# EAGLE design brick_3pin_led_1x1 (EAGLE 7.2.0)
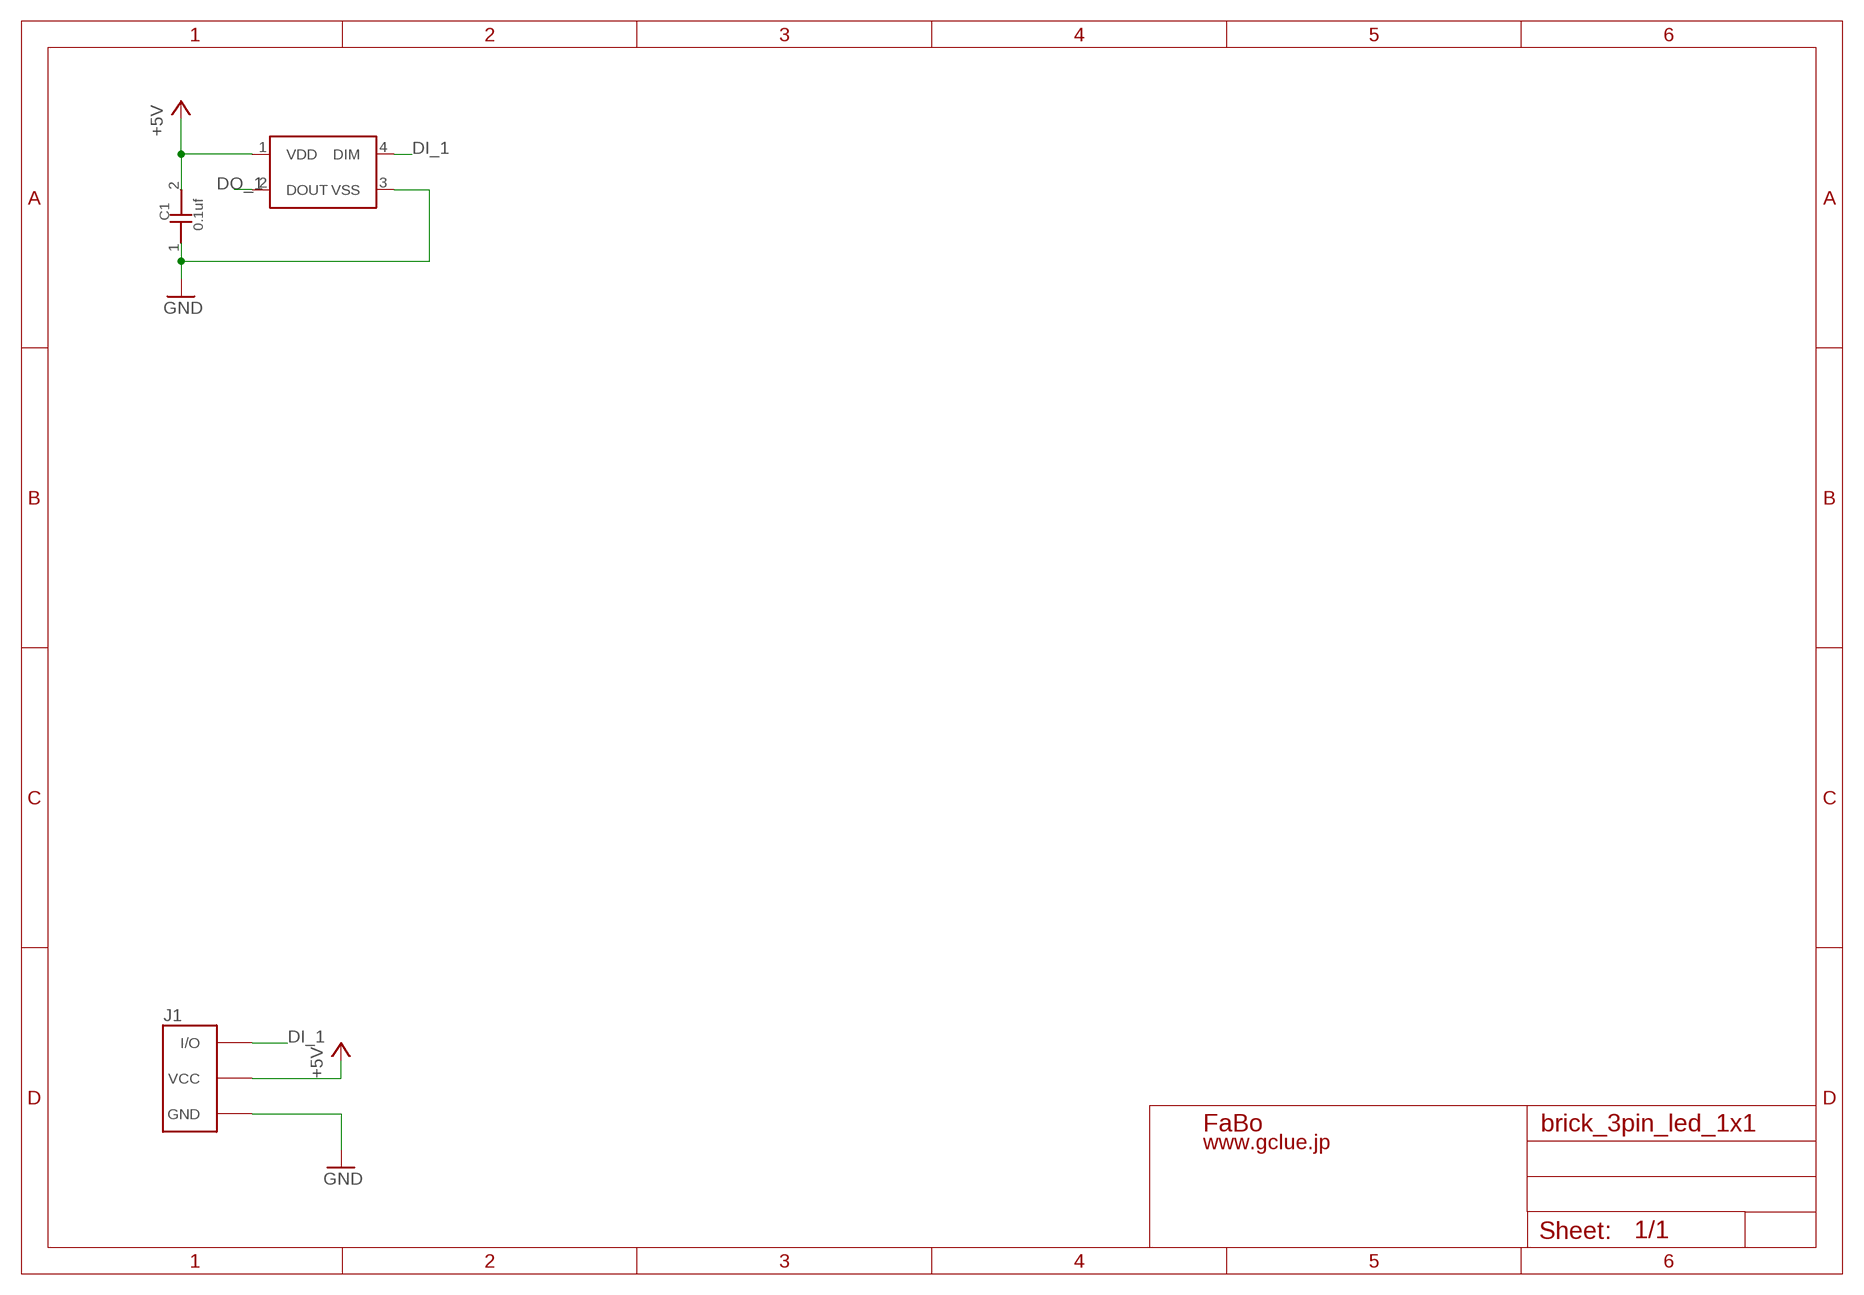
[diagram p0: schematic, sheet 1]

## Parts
C1  0.1uf  CAPACITOR0603  [0603]
J1  BRICK_3PIN  [BRICK_3PIN]
LED1  WS2818B  [WS2818B]

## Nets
+5V: C1.2 J1.VCC LED1.1(VDD)
DI_1: J1.IN/OUT(I/O) LED1.4(DIM)
DO_1: LED1.2(DOUT)
GND: C1.1 J1.GND LED1.3(VSS)

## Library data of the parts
C1 = GClue-Capacitor:CAPACITOR
J1 = GClue:BRICK_3PIN: FaBo Brick 3pin
LED1 = GClue-LED:WS2818B

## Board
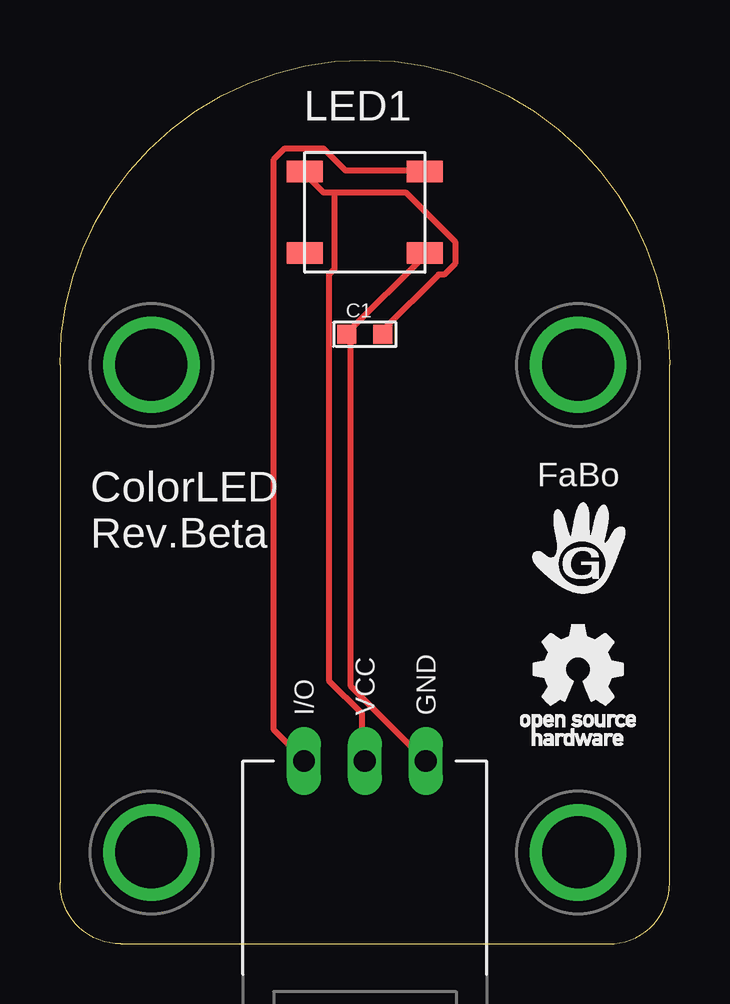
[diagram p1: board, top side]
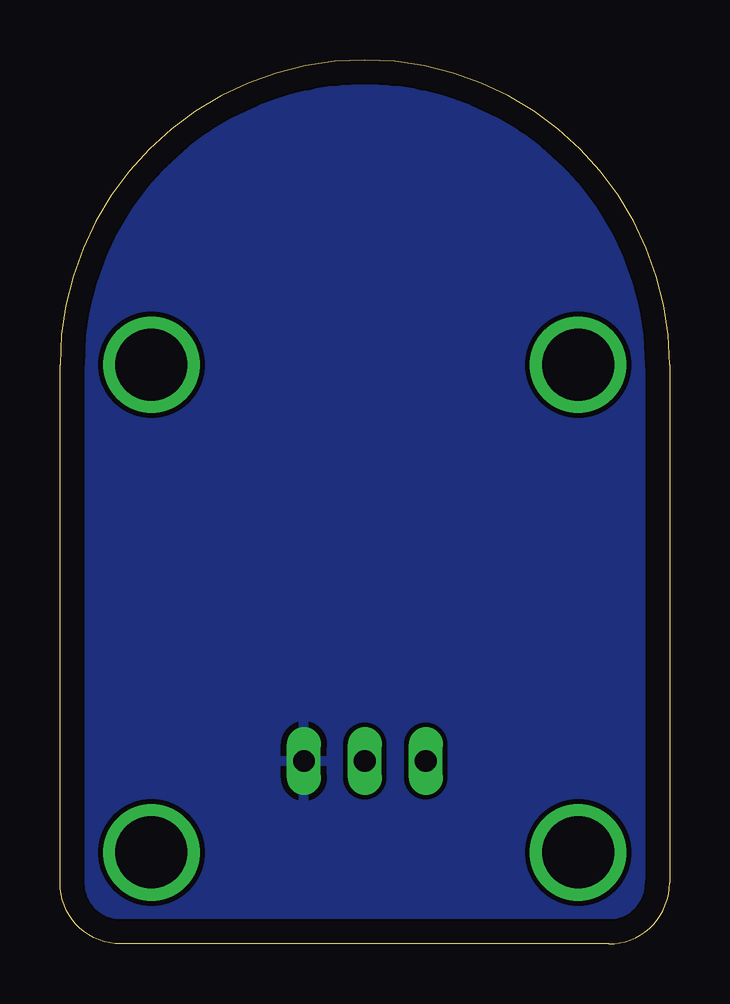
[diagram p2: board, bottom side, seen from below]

Size 25.4 x 36.83 mm. Coordinates in mm from the lower left corner, seen from the top.
Copper layers (1*16): Top 0.035mm / dielectric 1.5mm / Bottom 0.035mm
Design rules "default": minimum track width 10mil, minimum drill 24mil, track to track 8mil, track to pad 8mil, pad to pad 8mil, via to via 8mil, smd to smd 8mil, copper to edge 40mil, drill to drill 8mil, minimum pad ring 10mil, minimum via ring 8mil, stop-mask expansion 4mil, vias tented up to drill 0mil, thermal gap 10mil

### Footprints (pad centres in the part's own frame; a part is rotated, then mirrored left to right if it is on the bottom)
0603 = smd 0.8 x 0.8: 1 -0.75,0; 2 0.75,0
BRICK_3PIN = drill 0.9 long: GND 2.54,-10.16; IN/OUT -2.54,-10.16; VCC 0,-10.16 | drill 3 pad 3.81: P$5 -8.89,6.35; P$6 8.89,6.35; P$7 -8.89,-13.97; P$8 8.89,-13.97
WS2818B = smd 1.5 x 0.9: 1 -2.5,1.7; 2 -2.5,-1.7; 3 2.5,-1.7; 4 2.5,1.7

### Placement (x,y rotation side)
C1  12.7,25.4 0 top
J1  12.7,17.78 0 top
LED1  12.7,30.48 0 top
U$2  [LOGO_FABO_M]  21.59,16.51 0 top
U$3  [LOGO_OSHW_T_M]  21.59,11.43 0 top

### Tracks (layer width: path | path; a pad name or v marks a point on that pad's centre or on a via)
+5V
  Top 0.254: 11.43,31.32 10.97,31.32 10.29,32 LED1.1 | 11.43,31.32 14.4,31.32 16.46,29.26 16.46,28.35 16,27.89 15.77,27.89 13.49,25.6 C1.2 | 11.43,31.32 11.43,28.12 11.2,27.89 11.2,10.97 12.57,9.6 12.57,7.77 J1.VCC
DI_1
  Top 0.254: LED1.4 15.09,32.23 11.89,32.23 10.97,33.15 9.37,33.15 8.91,32.69 8.91,8.91 10.06,7.77 J1.IN/OUT
GND
  Top 0.254: LED1.3 15.09,28.57 12.12,25.6 C1.1 12.12,25.38 12.12,10.74 J1.GND
  pour Bottom: 0,0 25.4,0 25.4,36.83 0,36.83

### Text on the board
tPlace: ColorLED / Rev.Beta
